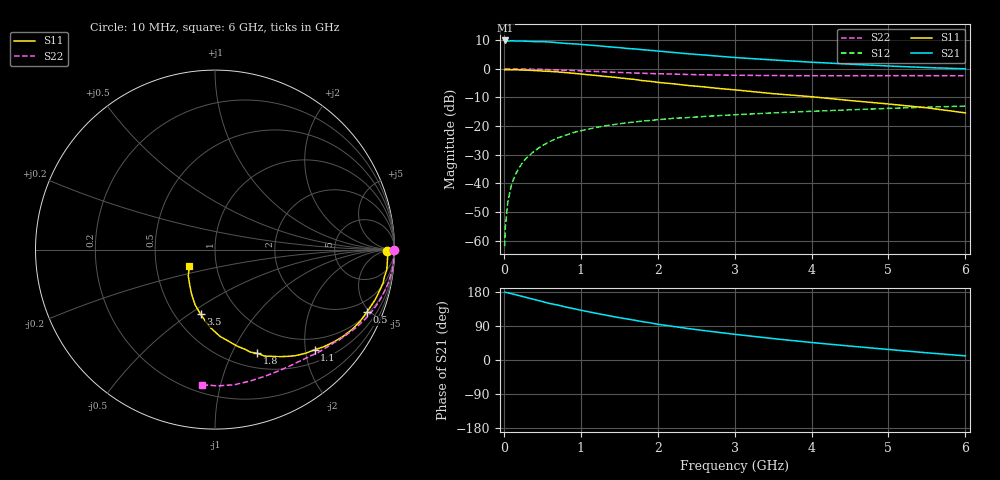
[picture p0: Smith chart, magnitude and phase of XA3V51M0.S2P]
! SIEMENS Discrete & RF Semiconductors
! BFY180
! Si NPN RF Bipolar Junction Transistor in MICRO-X
! VCE = 3.5 V  IC = 1 mA
! Common Emitter S-Parameters:  May  1997
# GHz  S  MA  R  50
!  f  S11  S21  S12  S22
! GHz  MAG  ANG  MAG  ANG  MAG  ANG  MAG  ANG
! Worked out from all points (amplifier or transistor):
!   36 points, 10 MHz to 6 GHz, reference 50 ohm
!   highest |S21| = 9.9 dB at 20 MHz (marker M1)
!   |S21| within 3 dB of that: start of sweep to 1.714 GHz
!   unconditionally stable (mu >= 1): 3.893 GHz to end of sweep
!   at 250 MHz: K = 0.09, MSG = 21.1 dB, |S12| = -32.5 dB
!   at 1.4 GHz: K = 0.50, MSG = 13.6 dB, |S12| = -19.6 dB
!   at 6 GHz: K = 1.06, MAG = 5.0 dB, |S12| = -13.0 dB
!   S11 on the Smith chart (normalised r, x): 10 MHz: 49, -8; 500 MHz: 1.12, -4.80; 1.1 GHz: 0.75, -2.19; 1.8 GHz: 0.67, -1.26; 3.5 GHz: 0.67, -0.56; 6 GHz: 0.74, -0.14
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0.01  0.9608 -0.4  3.079 179.5  0.0008 88.9  0.9988 -0.2
0.02  0.9657 -1.0  3.131 178.7  0.0017 94.4  0.9995 -0.5
0.05  0.9627 -2.1  3.05 177.5  0.0046 86.1  0.9966 -1.3
0.1  0.9628 -4.6  3.087 175.0  0.0095 87.5  0.9974 -2.7
0.15  0.9634 -6.9  3.06 172.5  0.0143 86.5  0.9971 -4.1
0.3  0.9477 -13.3  3.038 164.5  0.0282 80.8  0.9898 -8.0
0.5  0.915 -22.4  2.987 154.3  0.0456 74.6  0.9756 -13.1
0.6  0.9017 -26.3  2.942 148.9  0.0539 71.7  0.9667 -15.6
0.8  0.8614 -34.2  2.781 140.0  0.0692 66.1  0.9457 -20.2
1  0.8122 -41.8  2.679 131.4  0.0832 60.8  0.9227 -24.7
1.1  0.7871 -45.2  2.605 127.4  0.0884 58.3  0.91 -26.7
1.2  0.7662 -49.0  2.545 123.2  0.0947 56.0  0.899 -28.8
1.5  0.6967 -58.9  2.346 111.7  0.1098 50.3  0.8656 -34.2
1.8  0.6226 -67.9  2.161 101.3  0.1224 45.8  0.8367 -39.1
2  0.5807 -73.2  2.051 94.4  0.1294 42.7  0.8224 -42.2
2.2  0.5484 -77.5  1.935 88.7  0.1365 40.0  0.8108 -45.2
2.4  0.5108 -82.3  1.829 82.9  0.1413 37.8  0.7962 -48.0
2.8  0.4536 -90.6  1.66 72.7  0.1527 33.9  0.7792 -53.2
3.5  0.3689 -102.6  1.43 56.5  0.1701 27.8  0.7635 -62.1
4.5  0.2799 -117.8  1.207 36.7  0.1926 20.1  0.7579 -75.0
5.5  0.2087 -135.5  1.053 19.0  0.2142 12.3  0.7595 -88.8
6  0.1702 -147.1  1.001 10.9  0.2238 8.2  0.7563 -95.7
